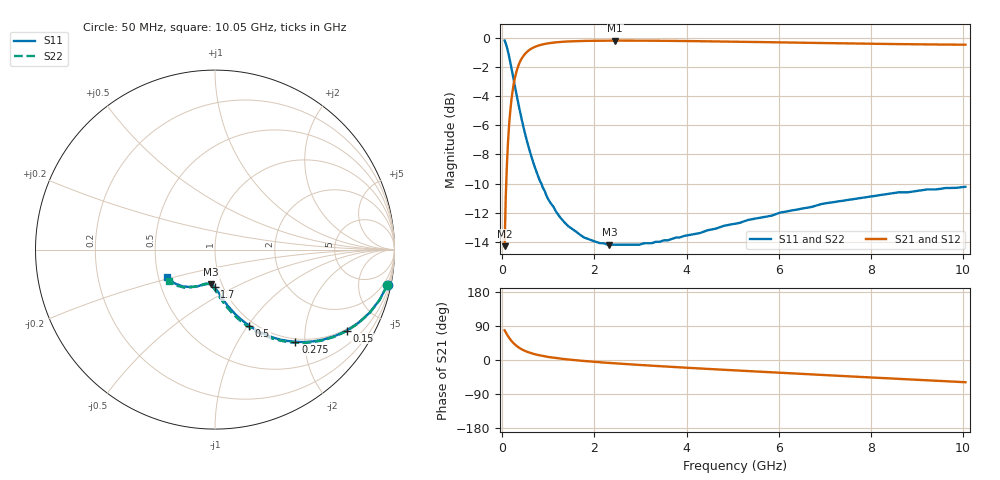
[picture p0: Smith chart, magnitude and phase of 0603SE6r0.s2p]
! AVX Thin Film Operation		Date: August 2001
! Description: Accu-P® Series, Thin Film, SMD, RF Capacitor
! Part Number: 06035J6R0BBT
! 50 MHz  -  10.05 GHz
! Serial Measurements
# mhz S db R 50
!	S11		S21		S12		S22
!	dB	Phase	dB	Phase	dB	Phase	dB	Phase
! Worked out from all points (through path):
!   401 points, 50 MHz to 10.05 GHz, reference 50 ohm
!   highest |S21| = -0.17 dB at 2.45 GHz (marker M1); lowest = -14.3 dB at 50 MHz (marker M2)
!   group delay of S21, straight-line fit = 22.7 ps
!   lowest |S11| = -14.2 dB at 2.325 GHz (marker M3), VSWR 1.48, Z = 44.5 - j17.9 ohm
!   |S11| at or under -10 dB: 847.8 MHz to end of sweep
!   |S22| runs from -14.2 to -0.2 dB; largest |S21 - S12| = 0
!   S11 on the Smith chart (normalised r, x): 50 MHz: 0.94, -9.84; 150 MHz: 0.94, -3.28; 275 MHz: 0.94, -1.81; 500 MHz: 0.94, -1.02; 1.7 GHz: 0.91, -0.40; 10.05 GHz: 0.55, -0.18
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50  -0.17 -11.5  -14.30 78.4  -14.30 78.4  -0.17 -11.6
100  -0.63 -22.3  -8.70 67.6  -8.70 67.6  -0.63 -22.5
125  -0.95 -27.2  -7.08 62.7  -7.08 62.7  -0.95 -27.4
150  -1.30 -31.6  -5.86 58.2  -5.86 58.2  -1.30 -32.0
200  -2.08 -39.5  -4.19 50.2  -4.19 50.2  -2.08 -40.0
275  -3.33 -48.9  -2.71 40.7  -2.71 40.7  -3.33 -49.6
325  -4.14 -53.9  -2.12 35.7  -2.12 35.7  -4.14 -54.6
375  -4.92 -58.0  -1.69 31.5  -1.69 31.5  -4.92 -58.9
500  -6.66 -65.8  -1.06 23.6  -1.06 23.6  -6.66 -66.9
600  -7.82 -70.2  -0.79 19.0  -0.79 19.0  -7.82 -71.6
700  -8.82 -73.7  -0.62 15.5  -0.62 15.5  -8.82 -75.2
1000  -11.10 -80.9  -0.36 8.0  -0.36 8.0  -11.10 -82.9
1325  -12.58 -86.0  -0.25 2.7  -0.25 2.7  -12.58 -88.3
1700  -13.54 -90.4  -0.20 -1.8  -0.20 -1.8  -13.54 -92.9
1725  -13.60 -90.7  -0.20 -2.1  -0.20 -2.1  -13.60 -93.2
2325  -14.20 -96.4  -0.18 -7.8  -0.18 -7.8  -14.20 -98.7
2450  -14.20 -97.5  -0.17 -8.9  -0.17 -8.9  -14.20 -99.8
3400  -14.00 -105.0  -0.19 -16.2  -0.19 -16.2  -14.00 -106.8
5050  -12.76 -117.4  -0.25 -27.4  -0.25 -27.4  -12.76 -117.4
6725  -11.60 -129.0  -0.33 -38.0  -0.33 -38.0  -11.50 -127.0
8400  -10.69 -140.1  -0.41 -48.6  -0.41 -48.6  -10.69 -136.2
10050  -10.22 -150.8  -0.46 -58.6  -0.46 -58.6  -10.20 -145.8
